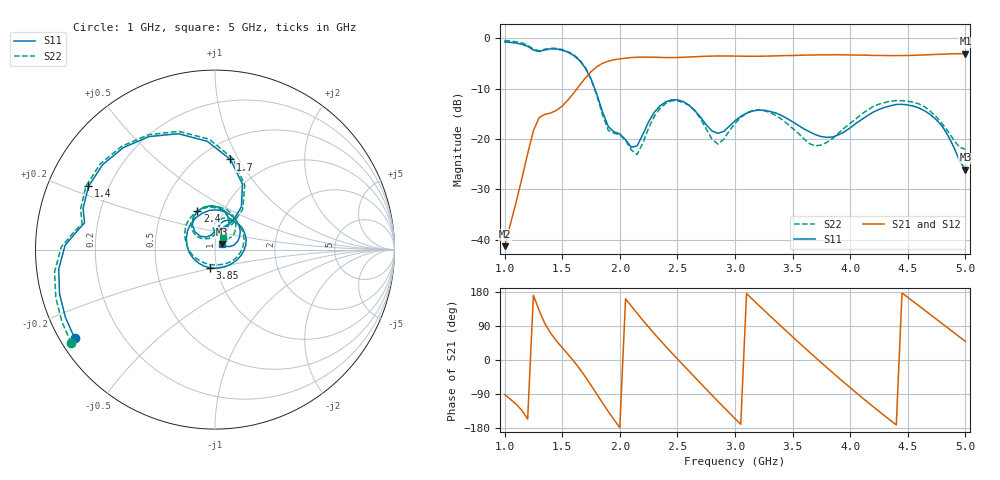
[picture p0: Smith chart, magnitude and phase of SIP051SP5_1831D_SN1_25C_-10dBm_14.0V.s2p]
# GHz  S  dB  R  50
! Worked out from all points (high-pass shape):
!   81 points, 1 GHz to 5 GHz, reference 50 ohm
!   highest |S21| = -3.01 dB at 5 GHz (marker M1); lowest = -41.3 dB at 1 GHz (marker M2)
!   |S21| within 3 dB of the highest: 1.78 GHz to end of sweep
!   lowest |S11| = -26.1 dB at 5 GHz (marker M3), VSWR 1.10, Z = 53.9 + j3.31 ohm
!   |S11| at or under -10 dB: 1.783 GHz to end of sweep
!   |S22| runs from -23.1 to -0.4 dB; largest |S21 - S12| = 0.0026
!   S11 on the Smith chart (normalised r, x): 1 GHz: 0.04, -0.29; 1.4 GHz: 0.13, +0.23; 1.7 GHz: 0.68, +0.92; 2.4 GHz: 0.75, +0.34; 3.85 GHz: 0.92, -0.19; 5 GHz: 1.08, +0.07
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1  -0.68 -147.8  -41.29 -91.1  -41.08 -90.6  -0.39 -146.9
1.25  -2.29 171.5  -18.34 170.8  -18.34 171.0  -2.10 172.1
1.4  -2.07 153.4  -14.82 70.7  -14.86 70.6  -1.93 153.9
1.55  -2.74 120.3  -12.23 15.1  -12.22 15.1  -2.62 120.1
1.7  -5.86 80.2  -7.88 -43.8  -7.89 -43.8  -5.74 78.8
1.85  -14.61 57.9  -4.94 -113.3  -4.93 -113.4  -15.20 55.6
2  -18.97 88.0  -4.05 -178.4  -4.05 -178.4  -19.14 88.2
2.2  -19.09 137.8  -3.71 104.8  -3.71 104.8  -20.79 139.2
2.35  -13.39 124.4  -3.76 52.1  -3.76 52.2  -13.88 130.4
2.4  -12.58 114.8  -3.79 35.4  -3.78 35.4  -12.89 119.8
2.55  -12.54 83.8  -3.73 -13.2  -3.74 -13.1  -12.70 86.0
2.75  -17.16 60.6  -3.53 -76.9  -3.52 -76.9  -17.96 58.0
3  -16.36 77.7  -3.50 -154.7  -3.48 -154.6  -16.88 91.7
3.15  -14.43 56.6  -3.53 160.7  -3.53 160.8  -14.32 65.8
3.35  -14.78 18.0  -3.46 103.3  -3.47 103.3  -15.25 20.2
3.5  -16.57 -12.8  -3.38 61.2  -3.37 61.2  -17.87 -20.1
3.7  -19.14 -59.4  -3.27 6.2  -3.27 6.3  -21.34 -88.2
3.85  -19.59 -106.5  -3.23 -33.9  -3.24 -34.0  -19.84 -140.2
4.1  -16.10 173.1  -3.30 -98.5  -3.30 -98.5  -15.02 159.9
4.35  -13.38 109.6  -3.40 -159.4  -3.41 -159.4  -12.46 111.4
4.7  -15.19 36.0  -3.20 118.9  -3.21 119.0  -14.55 52.1
5  -26.11 38.2  -3.01 49.0  -3.02 49.2  -22.01 57.3
